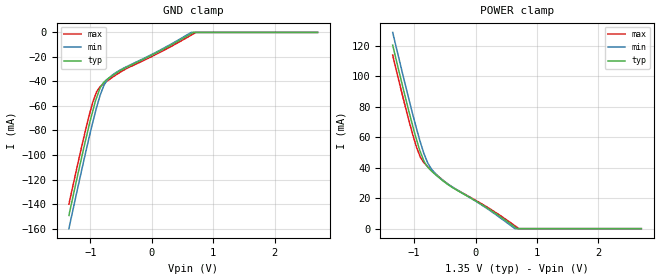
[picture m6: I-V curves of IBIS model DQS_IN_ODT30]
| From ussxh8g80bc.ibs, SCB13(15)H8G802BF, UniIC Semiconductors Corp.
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| MODEL DQS_IN_ODT30 (Data Strobe Input with 30ohm ODT, 800-2133Mbps)
[Model]   DQS_IN_ODT30
Model_type   Input
Vinl = 545.000mV
Vinh = 805.000mV
|   typ   min   max
|C_comp   1.105pF   1.047pF   1.139pF
C_comp_power_clamp   0.5525pF   0.5235pF   0.5695pF
C_comp_gnd_clamp   0.5525pF   0.5235pF   0.5695pF
| Note: C_comp changes when the ODT circuit is enabled.
[Model Spec]
| Input threshold voltage corners
Vinl   0.5450V   0.5115V   0.5825V
Vinh   0.8050V   0.7715V   0.8425V
| Dynamic Overshoot Parameters from DDR3L Specification
|D_overshoot_ampl_h   0.40   NA   NA
|D_overshoot_ampl_l   0.40   NA   NA
|D_overshoot_area_h   0.11n   NA   NA
|D_overshoot_area_l   0.11n   NA   NA
[Receiver Thresholds]
|Vth   =  0.675V
|Vth_min  =  0.6615V
|Vth_max  =  0.6885V
|Vinh_ac  =  0.130V
|Vinh_dc  =  0.090V
|Vinl_ac  = -0.130V
|Vinl_dc  = -0.090V
|Tslew_ac =  5.000ns |Not specified, so set to high value
|Threshold_sensitivity = 0.50
|Reference_supply Power_clamp_ref
|NOTE: If using the IBISCHK 4.2.1 or older parser, Differential receiver
|threshold parameters must be commented out because the parser generates
|errors for multiple differential models.
Vcross_low   = 0.545V
Vcross_high  = 0.805V
Vdiff_ac   = 260mV
Vdiff_dc   = 180mV
Tdiffslew_ac = 10.000ns |Not specified, so set to high value
[Voltage Range]   1.3500V   1.2830V   1.4250V
[POWER Clamp Reference]   1.3500V   1.2830V   1.4250V
| Junction Temperature (Ambient temp is 40C typ, 85C min, 0C max)
[Temperature Range]   45.0   90.0   0.0
[GND Clamp]
|   Voltage   I(typ)   I(min)   I(max)
-1.35V    -149.3mA   -160.1mA   -140.1mA
-1.085V   -89.13mA   -99.43mA   -80.74mA
-960mV    -63.79mA   -72.88mA   -56.68mA
-900mV    -53.32mA   -61.2mA    -48.47mA
-840mV    -45.08mA   -50.91mA   -44.12mA
-775mV    -40.35mA   -42.64mA   -41.41mA
-655mV    -35.63mA   -35.25mA   -37.1mA
-425mV    -28.77mA   -28.28mA   -29.84mA
65mV      -16.87mA   -16.28mA   -18.01mA
640mV     -1.008mA   -45.78uA   -2.27mA
720mV     0A         0A         0A
2.7V      0A         0A         0A
[POWER Clamp]
|   Voltage   I(typ)   I(min)   I(max)
-1.35V    120.3mA    128.6mA    113.7mA
-1.085V   76.62mA    84.61mA    70.66mA
-965mV    58.82mA    65.95mA    53.76mA
-900mV    50.41mA    56.66mA    46.88mA
-845mV    44.56mA    49.63mA    43.37mA
-775mV    40.18mA    42.71mA    40.42mA
-655mV    35.46mA    36.07mA    35.99mA
-525mV    31.14mA    31.44mA    31.52mA
200mV     13.25mA    12.84mA    13.82mA
640mV     1.022mA    41.43uA    1.907mA
705mV     0A         0A         0A
2.7V      0A         0A         0A
